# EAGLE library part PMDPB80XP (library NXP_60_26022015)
20 V, dual P-channel Trench MOSFET AAL Eindhoven MK
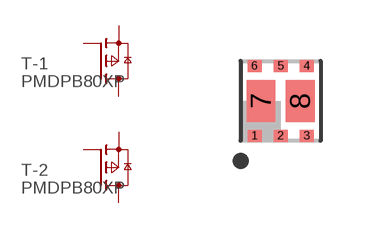
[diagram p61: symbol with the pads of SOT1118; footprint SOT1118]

Designator prefix T; gates -1=P-MOSFET_2D -2=P-MOSFET_2D

## PMDPB80XP  [SOT1118]
1  -1:S  pas
2  -1:G  pas
3  -2:D  pas
4  -2:S  pas
5  -2:G  pas
6  -1:D  pas
7  -1:D  pas
8  -2:D  pas

## Footprint SOT1118 (pad centres in mm)
SOT1118 HUSON6: plastic, thermal enhanced ultra thin small outline package; no leads;6 terminals; body 2 x 2 x 0.65 mm JEDEC: -- IEC: -- JEITA: --
smd 0.35 x 0.3: 1 -0.65,-0.875; 2 0,-0.875; 3 0.65,-0.875; 4 0.65,0.875; 5 0,0.875; 6 -0.65,0.875
smd 0.72 x 1.05: 7 -0.49,0; 8 0.49,0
